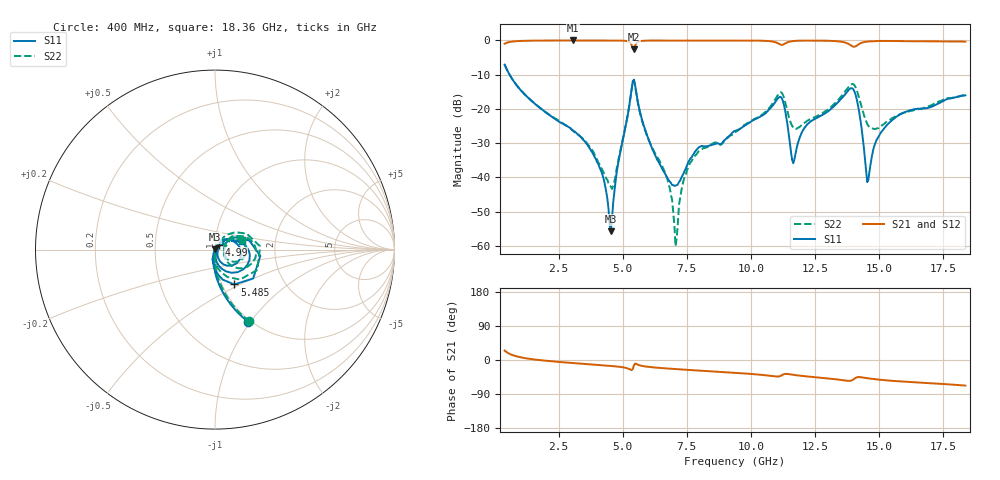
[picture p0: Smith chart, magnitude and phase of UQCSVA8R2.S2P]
!  Part Number  UQCSVA8R2.  Mounting Orientation: Horizontal
!  Description: Ultra Low ESR Microwave capacitors
!  Application: Coupling, Bypass, Tuning, DC Block
!  Filters, Matching
# GHZ S DB R 50
! Freq  |S11|  S11 Ph  |S21|  S21 Ph  |S12|  S12 Ph  |S22|  S22 Ph
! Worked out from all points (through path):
!   400 points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, 400 MHz to 18.36 GHz, reference 50 ohm
!   highest |S21| = -0.02 dB at 3.055 GHz (marker M1); lowest = -2.6 dB at 5.44 GHz (marker M2)
!   group delay of S21, straight-line fit = 11.2 ps
!   lowest |S11| = -55.8 dB at 4.54 GHz (marker M3), VSWR 1.00, Z = 49.9 + j0.133 ohm
!   |S11| at or under -10 dB: 592.2 MHz to end of sweep
!   |S22| runs from -60.1 to -7.1 dB; largest |S21 - S12| = 0.0036
!   S11 on the Smith chart (normalised r, x): 400 MHz: 0.97, -0.97; 4.99 GHz: 1.04, +0.05; 5.485 GHz: 1.14, -0.47; 18.36 GHz: 1.35, +0.13
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0.4  -7.08 -65.3  -0.97 24.8  -0.96 24.8  -7.06 -64.5
3.055  -26.24 -104.3  -0.02 -8.0  -0.01 -8.1  -26.34 -89.7
3.415  -28.62 -106.8  -0.03 -9.8  -0.02 -9.9  -28.43 -89.0
4.225  -39.57 -122.9  -0.03 -13.9  -0.02 -14.0  -38.04 -67.6
4.54  -55.75 125.0  -0.03 -15.7  -0.02 -15.8  -42.66 -14.4
4.99  -29.68 51.8  -0.08 -19.0  -0.08 -19.1  -29.29 62.1
5.44  -11.48 -37.1  -2.56 -14.0  -2.55 -14.1  -11.63 -25.7
5.485  -13.07 -61.0  -1.56 -9.6  -1.56 -9.7  -13.26 -50.1
6.385  -35.30 -100.5  -0.03 -20.6  -0.03 -20.7  -34.56 -86.0
6.835  -41.24 -83.2  -0.03 -22.9  -0.03 -23.0  -43.08 -93.0
7.06  -42.40 -49.1  -0.03 -23.9  -0.04 -24.0  -60.10 -150.0
7.195  -41.34 -22.3  -0.03 -24.5  -0.04 -24.6  -48.00 92.4
7.6  -34.98 20.9  -0.04 -26.3  -0.05 -26.4  -36.20 70.7
9.4  -26.38 37.2  -0.06 -33.8  -0.08 -33.9  -26.72 48.7
11.155  -16.53 -21.0  -1.25 -41.9  -1.25 -42.0  -15.16 -1.5
11.65  -35.88 -7.0  -0.19 -39.2  -0.20 -39.2  -25.55 -16.6
12.37  -23.45 51.0  -0.07 -44.5  -0.08 -44.5  -22.77 21.7
13.99  -14.31 -34.9  -1.84 -51.4  -1.84 -51.4  -12.78 -12.0
14.53  -41.39 -31.1  -0.35 -48.1  -0.36 -48.2  -24.41 -30.6
14.8  -30.93 43.6  -0.21 -50.4  -0.22 -50.4  -25.85 -1.6
15.385  -24.10 31.7  -0.16 -54.3  -0.17 -54.3  -23.39 30.1
18.355  -16.04 17.4  -0.38 -67.5  -0.39 -67.4  -15.87 18.9
